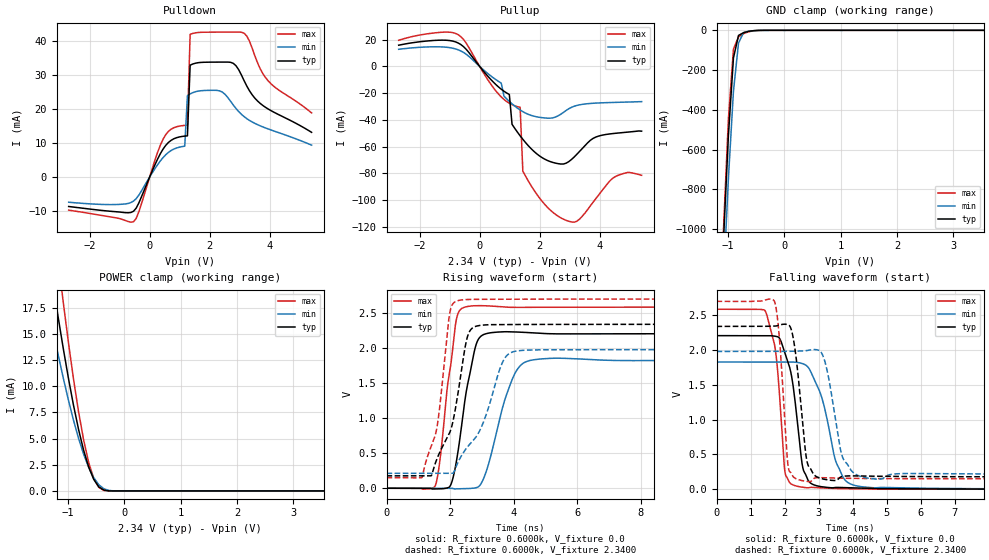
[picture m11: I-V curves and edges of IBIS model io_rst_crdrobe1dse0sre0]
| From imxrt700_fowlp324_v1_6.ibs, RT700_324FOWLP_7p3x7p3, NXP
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[Model] io_rst_crdrobe1dse0sre0
|   Model io_rst_crdrobe1dse0sre0
| This model was characterised for following simulation conditions:
| External (pad) voltage:
|   - Typ: 2.34V,   - Min: 1.98V,   - Max: 2.7V
| Library cells for typ/min/max conditions are connected as defined below:
|  PAD_RST - External Pad
|  ipp_do - Core Input
|  ipp_obe - Output Buffer Enable
|  ASRCN3V3[3] - NC
|  ASRCN3V3[4] - NC
|  ASRCP3V3[4] - NC
|  REFAPBIAS3V3 - gnde
|  REFBAMPL3V3 - vdd1v8
|  REFCAMPH3V3 - vdd1v8
|  REFDNBIAS3V3 - vdd1v8
|  REFH3V3 - REFH3V3
|  REFL3V3 - REFL3V3
|  gnde - gnde
|  ipp_dse - gnde
|  ipp_ina235_3v - NC
|  ipp_ina40_3v - NC
|  ipp_ina_mux - NC
|  ipp_ind - NC
|  ipp_ind_1p8v - NC
|  ipp_ind_3v - NC
|  ipp_sre - gnde
|  vdd - vdd
|  vdd1v8 - vdd1v8
|  vdda - vdde3v3
|  vdde3v3 - vdde3v3
| All other pins connected to ground
Model_type I/O
Polarity   Non-Inverting
Enable   Active-High
Vinl =   0.7020V
Vinh =   1.6300V
Vmeas =  1.1700V
Cref =   15.0000pF
Rref =   0.6000k
Vref =   0.0V
C_comp   3.9956pF   3.8199pF   4.1038pF
|C_comp_pullup   0.5142pF   0.5882pF   0.4996pF
|C_comp_pulldown   2.0717pF   2.1609pF   1.8543pF
[Model Spec]
| variable   typ   min   max
Vinh   1.6300V   NA   NA
Vinl   0.7020V   NA   NA
Vref   0.0V   0.0V   0.0V
Cref   15.0000pF   15.0000pF   15.0000pF
Rref   0.6000k   0.6000k   0.6000k
[Receiver Thresholds]
Vcross_high  =   0.0V
Vcross_low  =   0.0V
Vdiff_ac  =   0.0V
Vdiff_dc  =   0.0V
Tdiffslew_ac  =   0.0S
[Temperature Range]   25.0000   0.1250k   -40.0000
[Voltage Range]   2.3400V   1.9800V   2.7000V
[Pullup Reference]   2.3400V   1.9800V   2.7000V
[Pulldown Reference]   0.0V   0.0V   0.0V
[POWER Clamp Reference]   2.3400V   1.9800V   2.7000V
[GND Clamp Reference]   0.0V   0.0V   0.0V
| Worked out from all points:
|   slope of the pulldown table from 0 to 0.351 V, typ, clamps not added: 51.9 ohm
|   slope of the pullup table from 0 to 0.351 V, typ, clamps not added: 37.8 ohm
|   GND clamp passes 1 mA (typ) near -0.49 V on its own axis
|   POWER clamp passes 1 mA (typ) near -0.53 V on its own axis
|   rising waveform, R_fixture 0.6000k, V_fixture 0.0: 20-80 % time 458ps typ, 655ps min, 389ps max; typ from 0 V to 2.21 V
|   rising waveform, R_fixture 0.6000k, V_fixture 2.3400: 20-80 % time 656ps typ, 1.01ns min, 451ps max; typ from 0.177 V to 2.34 V
|   falling waveform, R_fixture 0.6000k, V_fixture 0.0: 20-80 % time 352ps typ, 554ps min, 257ps max; typ from 2.21 V to 0 V
|   falling waveform, R_fixture 0.6000k, V_fixture 2.3400: 20-80 % time 263ps typ, 360ps min, 204ps max; typ from 2.34 V to 0.177 V
[Pulldown]
|Voltage   I(typ)   I(min)   I(max)
-2.7V     -8.67mA    -7.41mA    -9.74mA
-450mV    -9.161mA   -6.365mA   -12.21mA
450mV     8.254mA    5.751mA    11.17mA
1.17V     12.03mA    9.072mA    15.18mA
1.26V     12.11mA    23.94mA    15.24mA
1.35V     32.9mA     24.45mA    41.96mA
2.34V     33.8mA     25.32mA    42.61mA
2.79V     33.43mA    21.16mA    42.62mA
3.15V     28.33mA    17.76mA    42.29mA
3.51V     23.17mA    15.76mA    35.6mA
3.96V     19.96mA    14.11mA    28.19mA
5.4V      13.14mA    9.377mA    18.85mA
[Pullup]
|Voltage   I(typ)   I(min)   I(max)
-2.7V     15.88mA    12.82mA    19.56mA
-540mV    14.85mA    10.51mA    20.28mA
720mV     -17.09mA   -12.5mA    -22.86mA
990mV     -21.04mA   -26.21mA   -27.62mA
1.08V     -43.37mA   -28.03mA   -28.69mA
1.35V     -52.01mA   -32.66mA   -30.61mA
1.44V     -54.61mA   -33.9mA    -78.45mA
2.7V      -73.13mA   -35.9mA    -113.4mA
3.24V     -65.84mA   -29.25mA   -116mA
3.87V     -52.96mA   -27.49mA   -99.18mA
4.5V      -50.17mA   -26.97mA   -82.85mA
5.4V      -48.51mA   -26.38mA   -81.57mA
[GND_clamp]
|Voltage   I(typ)   I(min)   I(max)
-2.7V     -12.91A    -12.88A    -13.56A
-1.08V    -1.077A    -1.286A    -1.025A
-990mV    -533.6mA   -749.4mA   -449.1mA
-900mV    -139.2mA   -307mA     -94.25mA
-810mV    -25.49mA   -63.91mA   -32.87mA
-720mV    -11.78mA   -11.41mA   -16.65mA
-540mV    -1.684mA   -1.901mA   -2.149mA
-360mV    -36.04uA   -133.3uA   -15.05uA
5.4V      0A         0A         0A
[POWER_clamp]
|Voltage   I(typ)   I(min)   I(max)
-2.7V     73.96mA    57.58mA    95.4mA
-1.44V    26.15mA    20.18mA    34.67mA
-1.35V    22.86mA    17.7mA     30.34mA
-1.26V    19.66mA    15.3mA     26.09mA
-1.17V    16.56mA    12.98mA    21.97mA
-1.08V    13.59mA    10.78mA    17.99mA
-900mV    8.212mA    6.776mA    10.73mA
-720mV    3.9mA      3.518mA    4.888mA
-630mV    2.284mA    2.252mA    2.724mA
-540mV    1.103mA    1.268mA    1.195mA
-360mV    77.93uA    204.3uA    41.52uA
5.4V      0A         0A         0A
[Ramp]
| variable   typ   min   max
dV/dt_r  1.3244/0.4580n   1.0971/0.6554n   1.5519/0.3886n
dV/dt_f  1.2978/0.2633n   1.0605/0.3602n   1.5299/0.2037n
R_load = 0.6000k
[Rising Waveform]
R_fixture= 0.6000k
V_fixture= 0.0
V_fixture_min= 0.0
V_fixture_max= 0.0
|time   V(typ)   V(min)   V(max)
0s        133.2nV    3.451uV    44.06nV
1.533ns   -9.472mV   -1.02mV    33.95mV
1.689ns   -8.419mV   -1.151mV   421.3mV
1.988ns   22.41mV    -654.7uV   1.665V
2.2ns     379.3mV    -8.557mV   2.408V
2.679ns   1.761V     -1.51mV    2.602V
3.098ns   2.2V       184.1mV    2.604V
4.063ns   2.23V      1.655V     2.581V
4.94ns    2.208V     1.848V     2.583V
60ns      2.207V     1.829V     2.586V
[Rising Waveform]
R_fixture= 0.6000k
V_fixture= 2.3400
V_fixture_min= 1.9800
V_fixture_max= 2.7000
|time   V(typ)   V(min)   V(max)
0s        177mV      212.5mV    150.2mV
1.122ns   176.2mV    212.4mV    156.7mV
1.409ns   179.2mV    212mV      602.5mV
1.589ns   420.5mV    211.6mV    866.8mV
2.006ns   812.1mV    212.9mV    2.534V
2.406ns   1.821V     498.9mV    2.689V
2.747ns   2.299V     691.5mV    2.696V
3.712ns   2.337V     1.847V     2.698V
4.339ns   2.337V     1.969V     2.699V
60ns      2.34V      1.98V      2.7V
[Falling Waveform]
R_fixture= 0.6000k
V_fixture= 0.0
V_fixture_min= 0.0
V_fixture_max= 0.0
|time   V(typ)   V(min)   V(max)
0s        2.207V     1.828V     2.586V
1.424ns   2.208V     1.828V     2.566V
1.711ns   2.2V       1.828V     2.059V
1.856ns   2.164V     1.827V     1.32V
2.027ns   1.929V     1.829V     206.2mV
2.513ns   366.1mV    1.807V     29.52mV
2.667ns   149.1mV    1.766V     19.29mV
3.718ns   22.49mV    170.2mV    7.143mV
4.618ns   9.952mV    19.87mV    2.453mV
60ns      2.991uV    16.17uV    1.714uV
[Falling Waveform]
R_fixture= 0.6000k
V_fixture= 2.3400
V_fixture_min= 1.9800
V_fixture_max= 2.7000
|time   V(typ)   V(min)   V(max)
0s        2.34V      1.98V      2.7V
1.702ns   2.344V     1.98V      2.7V
1.851ns   2.36V      1.979V     2.145V
2.107ns   2.362V     1.981V     314.7mV
2.287ns   2.077V     1.983V     164mV
2.692ns   341.3mV    1.996V     109.3mV
3.154ns   143.1mV    1.881V     164.5mV
3.735ns   185.8mV    423.7mV    157mV
4.677ns   186.1mV    145.4mV    152.4mV
60ns      177mV      212.6mV    150.2mV
